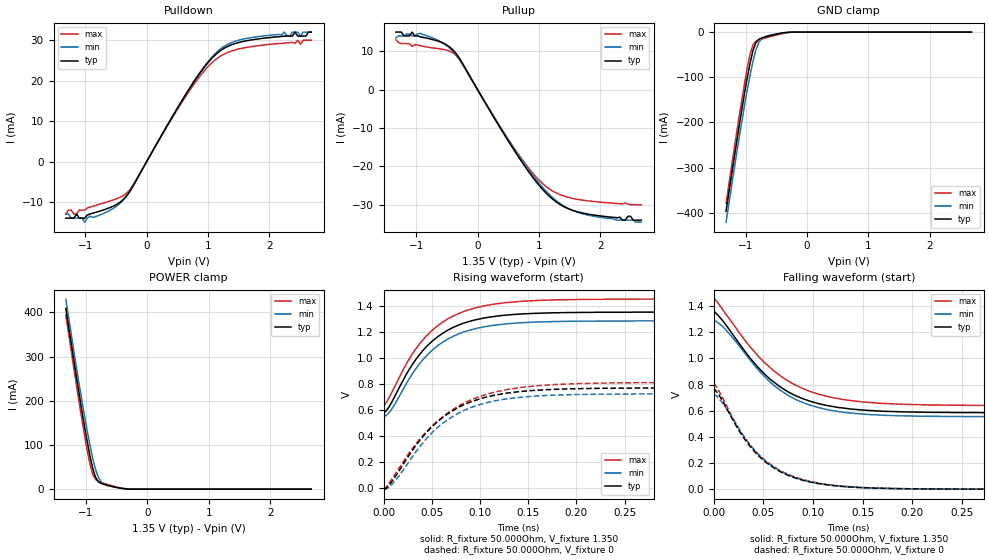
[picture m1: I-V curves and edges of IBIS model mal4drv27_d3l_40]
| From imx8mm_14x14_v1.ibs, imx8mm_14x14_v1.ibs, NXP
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[Model] mal4drv27_d3l_40
Model_type   I/O
Polarity   Non-Inverting
Enable   Active-High
C_comp   1.534pF   1.526pF   1.541pF
C_comp_pullup   672.952fF   657.747fF   679.061fF
C_comp_pulldown 805.206fF   796.471fF   820.214fF
Vinh = 805.000mV
Vinl = 545.000mV
Vmeas = 675.000mV
Vref = 675.000mV
Rref = 50Ohms
Cref = 0pF
[Model Spec]
Vinh   805.000mV   772.000mV   855.000mV
Vinl   545.000mV   512.000mV   595.000mV
Vmeas   675.000mV   642.000mV   725.000mV
Vref   675.000mV   642.000mV   725.000mV
D_overshoot_ampl_h 0.4 NA   NA
D_overshoot_ampl_l 0.4 NA   NA
D_overshoot_area_l 110.000m NA   NA
D_overshoot_area_h 110.000m NA   NA
|[Receiver Thresholds]
|Vth = 675.000mV
|Vth_min = 642.000mV
|Vth_max = 725.000mV
|Vinh_ac = 150.000mV
|Vinh_dc = 100.000mV
|Vinl_ac = -150.000mV
|Vinl_dc = -100.000mV
|Tslew_ac = 5.000ns
|Threshold_sensitivity = 0.5
|Reference_supply Pullup_ref
[Temperature Range]   25.000   125.000   -40.000
[Voltage Range]   1.350V   1.283V   1.450V
[GND Clamp Reference]   0.00V   0.00V   0.00V
|[C Comp Corner]
|| variable   typ   min   max
|C_comp 1.541pF   1.526pF   1.534pF
|C_comp_pullup 679.061fF   657.747fF   672.952fF
|C_comp_pulldown 805.206fF   820.214fF   796.471fF
[Pulldown Reference]   0.00V   0.00V   0.00V
[POWER Clamp Reference]   1.350V   1.283V   1.450V
[Pullup Reference]   1.350V   1.283V   1.450V
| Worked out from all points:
|   slope of the pulldown table from 0 to 0.203 V, typ, clamps not added: 37.2 ohm
|   slope of the pullup table from 0 to 0.203 V, typ, clamps not added: 36.6 ohm
|   GND clamp passes 1 mA (typ) near -0.34 V on its own axis
|   POWER clamp passes 1 mA (typ) near -0.37 V on its own axis
|   rising waveform, R_fixture 50.000Ohm, V_fixture 1.350: 20-80 % time 49.3ps typ, 49.3ps min, 51.4ps max; typ from 0.581 V to 1.35 V
|   rising waveform, R_fixture 50.000Ohm, V_fixture 0: 20-80 % time 59ps typ, 57.7ps min, 65.7ps max; typ from -0.004 V to 0.77 V
|   falling waveform, R_fixture 50.000Ohm, V_fixture 1.350: 20-80 % time 58.8ps typ, 57.7ps min, 63.8ps max; typ from 1.35 V to 0.585 V
|   falling waveform, R_fixture 50.000Ohm, V_fixture 0: 20-80 % time 49.3ps typ, 49.6ps min, 50.4ps max; typ from 0.771 V to 0 V
[GND Clamp]
-1.318V   -397mA     -421mA     -379mA
-1.099V   -203mA     -229mA     -182mA
-1.011V   -130mA     -157mA     -109mA
-966.7mV  -96.76mA   -124mA     -75.62mA
-922.7mV  -66.15mA   -92.44mA   -47.23mA
-878.8mV  -40.87mA   -64.33mA   -28.32mA
-834.8mV  -24.17mA   -41.16mA   -20.75mA
-790.9mV  -16.5mA    -24.84mA   -17.97mA
-747mV    -13.39mA   -15.69mA   -16.02mA
-571.2mV  -6.876mA   -6.005mA   -9.023mA
-219.7mV  -49.34uA   -80.18uA   -119uA
2.68V     51.21nA    1.31uA     23.01nA
[Power Clamp]
-1.33V    409mA      430mA      393.3mA
-1.111V   214mA      236.6mA    194.7mA
-1.023V   140mA      164.6mA    120.2mA
-934.8mV  73.93mA    98.06mA    55.78mA
-890.9mV  46.71mA    69.56mA    33.54mA
-847mV    27.2mA     45.54mA    22.2mA
-803mV    17.25mA    27.9mA     17.76mA
-759.1mV  13.27mA    17.3mA     15.42mA
-715.2mV  11.13mA    11.9mA     13.45mA
-539.4mV  4.955mA    4.74mA     6.349mA
-275.8mV  101uA      270.7uA    142.8uA
2.668V    -162nA     -1.898uA   -65.08nA
[Pulldown]
-1.318V   -14mA      -13mA      -13mA
-1.274V   -14mA      -13mA      -12mA
-1.142V   -13mA      -14mA      -13mA
-1.011V   -14mA      -15mA      -12mA
-395.5mV  -9.582mA   -9.747mA   -8.551mA
-219.7mV  -5.977mA   -5.954mA   -5.802mA
747mV     19.2mA     19.28mA    18.63mA
1.011V    24.67mA    24.92mA    23.67mA
1.23V     27.7mA     28.16mA    26.31mA
1.67V     29.98mA    30.56mA    28.33mA
2.592V    31mA       32mA       30mA
2.68V     32mA       32mA       30mA
[Pullup]
-1.33V    15mA       13.53mA    13mA
-1.199V   14mA       14mA       12mA
-1.067V   15mA       14mA       11.28mA
-934.8mV  13.78mA    14.7mA     11.43mA
-583.3mV  12.29mA    12.33mA    10.56mA
-407.6mV  10.46mA    10.12mA    9.639mA
-275.8mV  7.672mA    7.419mA    7.383mA
734.8mV   -19.14mA   -18.69mA   -18.4mA
998.5mV   -24.83mA   -24.31mA   -23.53mA
1.262V    -29.02mA   -28.66mA   -26.76mA
1.746V    -32.25mA   -32.48mA   -28.86mA
2.668V    -34mA      -34.53mA   -30mA
[Ramp]
R_load=50.000Ohm
dV/dt_r   460.500mV/55.000ps  436.198mV/55.000ps  486.300mV/59.500ps
dV/dt_f   460.500mV/55.000ps  436.199mV/55.000ps  486.300mV/57.500ps
[Rising waveform]
R_fixture=50.000Ohm
V_fixture=1.350
V_fixture_min=1.283
V_fixture_max=1.450
0s        581mV      550mV      631mV
7ps       642mV      593mV      714mV
25ps      892mV      822mV      973mV
36ps      1.014V     943mV      1.095V
45ps      1.09V      1.02V      1.173V
68ps      1.218V     1.15V      1.304V
98ps      1.295V     1.228V     1.388V
128ps     1.328V     1.26V      1.424V
177ps     1.345V     1.278V     1.444V
470ps     1.35V      1.283V     1.45V
[Rising waveform]
R_fixture=50.000Ohm
V_fixture=0
0s        -3.814mV   -3.021mV   -5.299mV
4ps       11.77mV    2.066mV    23.37mV
12ps      90.21mV    60.21mV    113mV
34ps      336mV      286mV      347mV
57ps      519mV      474mV      525mV
83ps      640mV      597mV      652mV
117ps     716mV      673mV      741mV
158ps     752mV      708mV      786mV
206ps     765mV      720mV      804mV
471ps     770mV      725mV      811mV
[Falling waveform]
R_fixture=50.000Ohm
V_fixture=1.350
V_fixture_min=1.283
V_fixture_max=1.450
0s        1.355V     1.285V     1.454V
6ps       1.316V     1.264V     1.405V
14ps      1.238V     1.204V     1.32V
37ps      999mV      984mV      1.085V
59ps      827mV      804mV      914mV
83ps      713mV      684mV      793mV
116ps     637mV      606mV      706mV
150ps     605mV      574mV      667mV
199ps     590mV      559mV      647mV
470ps     585mV      554mV      640mV
[Falling waveform]
R_fixture=50.000Ohm
V_fixture=0
0s        771mV      727mV      812mV
10ps      659mV      648mV      681mV
27ps      429mV      442mV      442mV
46ps      249mV      258mV      260mV
57ps      181mV      186mV      190mV
70ps      123mV      126mV      131mV
98ps      53.29mV    54.43mV    57.87mV
132ps     19.48mV    19.26mV    21.45mV
170ps     6.274mV    6.095mV    6.946mV
469ps     14.01uV    18.3uV     15.39uV
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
